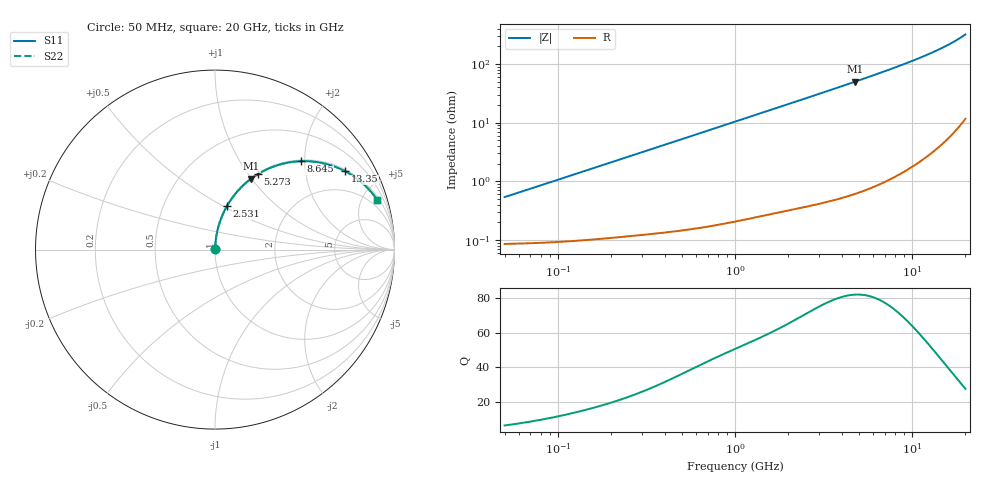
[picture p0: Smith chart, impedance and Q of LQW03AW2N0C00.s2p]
!Murata Part Number: LQW03AW2N0C00
!These Parameters are Measured in Series Mode Connection
!  o--[Z]--o
!Port1  Port2
!  o-------o
!Freq. Start=50[MHz] Stop=20[GHz], 401[Steps]
# Hz S RI R 50
!Freq.(Hz) S11(Real) S11(Imag) S21(Real) S21(Imag) S12(Real) S12(Imag) S22(Real) S22(Imag)
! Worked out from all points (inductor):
!   401 points, 50 MHz to 20 GHz, reference 50 ohm
!   read as one part in series: L = 1.69 nH near 51.52 MHz
!   highest Q = 82.1 at 4.748 GHz (marker M1), where L = 1.67 nH
!   S11 on the Smith chart (normalised r, x): 50 MHz: 1.00, +0.01; 2.531 GHz: 1.01, +0.53; 5.273 GHz: 1.01, +1.11; 8.645 GHz: 1.03, +1.91; 13.35 GHz: 1.07, +3.27; 20 GHz: 1.23, +6.40
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5e7  0.000885 0.00532  0.9991 -0.00532  0.9991 -0.00532  0.000885 0.00532
1.364002e8  0.00119 0.0144  0.9988 -0.0144  0.9988 -0.0144  0.00119 0.0144
3.721004e8  0.00282 0.0389  0.9972 -0.0389  0.9972 -0.0389  0.00282 0.0389
6.285508e8  0.00588 0.0652  0.9941 -0.0652  0.9941 -0.0652  0.00588 0.0652
1e9  0.0127 0.1027  0.9873 -0.1027  0.9873 -0.1027  0.0127 0.1027
1.614971e9  0.03 0.1624  0.97 -0.1624  0.97 -0.1624  0.03 0.1624
2.05233e9  0.0463 0.2027  0.9537 -0.2027  0.9537 -0.2027  0.0463 0.2027
2.531158e9  0.0678 0.2444  0.9322 -0.2444  0.9322 -0.2444  0.0678 0.2444
2.728004e9  0.0776 0.2608  0.9224 -0.2608  0.9224 -0.2608  0.0776 0.2608
3.626126e9  0.1285 0.3284  0.8715 -0.3284  0.8715 -0.3284  0.1285 0.3284
4.748272e9  0.2027 0.396  0.7973 -0.396  0.7973 -0.396  0.2027 0.396
5.273168e9  0.2398 0.4209  0.7602 -0.4209  0.7602 -0.4209  0.2398 0.4209
6.217679e9  0.308 0.4555  0.692 -0.4555  0.692 -0.4555  0.308 0.4555
7.442007e9  0.3956 0.4824  0.6044 -0.4824  0.6044 -0.4824  0.3956 0.4824
8.644534e9  0.4769 0.4924  0.5231 -0.4924  0.5231 -0.4924  0.4769 0.4924
9.745021e9  0.5454 0.4903  0.4546 -0.4903  0.4546 -0.4903  0.5454 0.4903
1.082228e10  0.6061 0.4804  0.3939 -0.4804  0.3939 -0.4804  0.6061 0.4804
1.201863e10  0.666 0.4626  0.334 -0.4626  0.334 -0.4626  0.666 0.4626
1.334722e10  0.7236 0.4372  0.2764 -0.4372  0.2764 -0.4372  0.7236 0.4372
1.621653e10  0.8202 0.3714  0.1798 -0.3714  0.1798 -0.3714  0.8202 0.3714
1.855685e10  0.8762 0.3139  0.1238 -0.3139  0.1238 -0.3139  0.8762 0.3139
2e10  0.9028 0.2786  0.0972 -0.2786  0.0972 -0.2786  0.9028 0.2786
